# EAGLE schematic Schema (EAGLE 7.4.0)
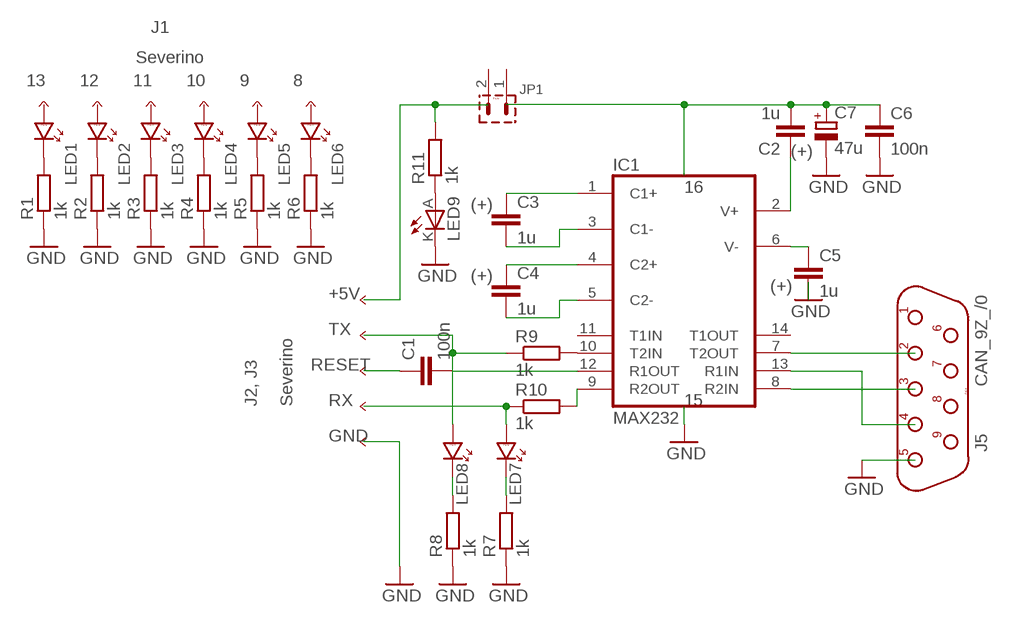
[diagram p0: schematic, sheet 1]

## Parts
C1  100n  KERAMICKYRM5  [KERAMICKY_RM5]
C2  1u  FOLIOVYRM5/4,5-7,2  [FOLIOVY_RM5/4,5-7,2]
C3  1u  FOLIOVYRM5/4,5-7,2  [FOLIOVY_RM5/4,5-7,2]
C4  1u  FOLIOVYRM5/4,5-7,2  [FOLIOVY_RM5/4,5-7,2]
C5  1u  FOLIOVYRM5/4,5-7,2  [FOLIOVY_RM5/4,5-7,2]
C6  100n  KERAMICKYRM5  [KERAMICKY_RM5]
C7  47u  ELEKTROLITICKYRM3,5-8  [ELEKTROLITICKY_RM3,5-8]
IC1  MAX232  [DIL16]
J5  CAN_9Z_/0  [CAN9Z]
JP1  PSH02-02P  [PSH02-02P]
LED1  LED_2,5X5  [LED2,5X5]
LED2  LED_2,5X5  [LED2,5X5]
LED3  LED_2,5X5  [LED2,5X5]
LED4  LED_2,5X5  [LED2,5X5]
LED5  LED_2,5X5  [LED2,5X5]
LED6  LED_2,5X5  [LED2,5X5]
LED7  LED_2,5X5  [LED2,5X5]
LED8  LED_2,5X5  [LED2,5X5]
LED9  LEDLED3MM  [LED3MM]
R1  1k  R-EU_0204/7  [0204/7]
R2  1k  R-EU_0204/7  [0204/7]
R3  1k  R-EU_0204/7  [0204/7]
R4  1k  R-EU_0204/7  [0204/7]
R5  1k  R-EU_0204/7  [0204/7]
R6  1k  R-EU_0204/7  [0204/7]
R7  1k  R-EU_0204/7  [0204/7]
R8  1k  R-EU_0204/7  [0204/7]
R9  1k  R-EU_0204/7  [0204/7]
R10  1k  R-EU_0204/7  [0204/7]
R11  1k  R-EU_0204/7  [0204/7]

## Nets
GND: C5.P$2 C6.P$2 C7.P$1(-) J5.5 LED9.K(C) R1.1 R2.1 R3.1 R4.1 R5.1 R6.1 R7.1 R8.1
N$1: C3.P$1 IC1.1(C1+)
N$2: C3.P$2 IC1.3(C1-)
N$3: C2.P$1 IC1.2(V+)
N$4: C4.P$1 IC1.4(C2+)
N$5: C4.P$2 IC1.5(C2-)
N$6: C5.P$1 IC1.6(V-)
N$7: C1.P$2 IC1.12(R1OUT)
N$8: IC1.9(R2OUT) R10.2
N$9: IC1.10(T2IN) R9.2
N$10: LED8.A R9.1
N$11: LED7.A R10.1
N$12: LED8.K R8.2
N$13: LED7.K R7.2
N$14: IC1.7(T2OUT) J5.2
N$15: IC1.8(R2IN) J5.3
N$16: IC1.13(R1IN) J5.4
N$17: C1.P$1
N$18: C2.P$2 C6.P$1 C7.P$2(+)
N$19: LED9.A R11.1
N$20: LED1.K R1.2
N$22: LED2.K R2.2
N$24: LED3.K R3.2
N$26: LED4.K R4.2
N$28: LED5.K R5.2
N$30: LED6.K R6.2
N$32: R11.2
Unconnected: IC1.11(T1IN) IC1.14(T1OUT) J5.1 J5.6 J5.7 J5.8 J5.9 JP1.1 JP1.2 LED1.A LED2.A LED3.A LED4.A LED5.A LED6.A

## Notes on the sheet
- J1
- Severino
- 13 | 12 | 11 | 10 | 9 | 8
- (+)
- 16
- (+)
- (+)
- (+)
- +5V
- TX
- RESET
- J2, J3 | Severino | RX | 15
- GND

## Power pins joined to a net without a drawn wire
GND: IC1.15(GND)
VCC: IC1.16(VCC)

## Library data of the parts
C1 C6 = #Kondenzatory:KERAMICKY
C2-C5 = #Kondenzatory:FOLIOVY
C7 = #Kondenzatory:ELEKTROLITICKY
IC1 = maxim:MAX232: RS232 TRANSCEIVER; MF: MAXIM; MPN: MAX232ACPE+; OC_FARNELL: 9723773; OC_NEWARK: 68K4544
J5 = #PaJa_konektory:CAN_9Z: Konektory CANNON - zasuvka - 9pinu
JP1 = #PaJa_konektory:PSH02-02: Konektory se zamkem - vidlice - 2pin
LED1-LED8 = #PaJa_31:LED: LED - jednobarevna
LED9 = #Led:LED
R1-R11 = #Odpory:R-EU_: RESISTOR, European symbol

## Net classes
1 power: width 0.61 mm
